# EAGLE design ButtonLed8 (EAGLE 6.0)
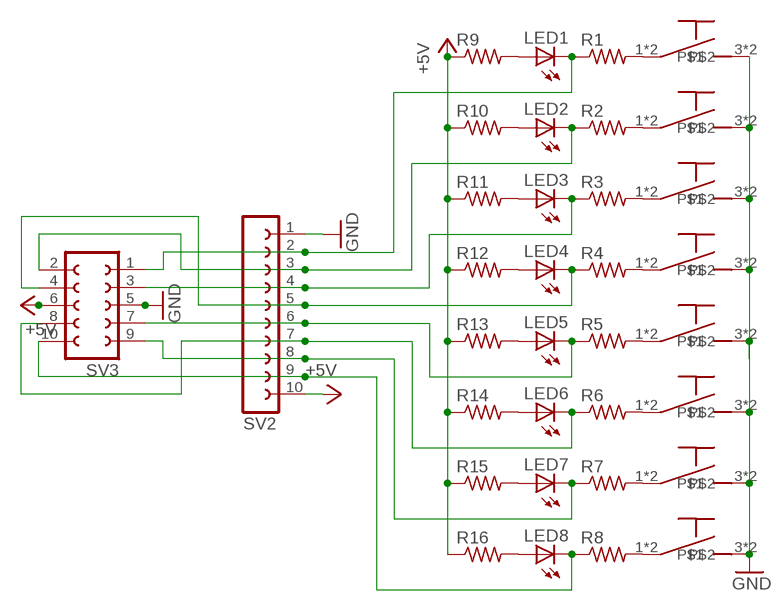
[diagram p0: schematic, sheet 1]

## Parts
LED1  LED3MM  [LED3MM]
LED2  LED3MM  [LED3MM]
LED3  LED3MM  [LED3MM]
LED4  LED3MM  [LED3MM]
LED5  LED3MM  [LED3MM]
LED6  LED3MM  [LED3MM]
LED7  LED3MM  [LED3MM]
LED8  LED3MM  [LED3MM]
R1  R-US_0204/7  [0204/7]
R2  R-US_0204/7  [0204/7]
R3  R-US_0204/7  [0204/7]
R4  R-US_0204/7  [0204/7]
R5  R-US_0204/7  [0204/7]
R6  R-US_0204/7  [0204/7]
R7  R-US_0204/7  [0204/7]
R8  R-US_0204/7  [0204/7]
R9  R-US_0204/7  [0204/7]
R10  R-US_0204/7  [0204/7]
R11  R-US_0204/7  [0204/7]
R12  R-US_0204/7  [0204/7]
R13  R-US_0204/7  [0204/7]
R14  R-US_0204/7  [0204/7]
R15  R-US_0204/7  [0204/7]
R16  R-US_0204/7  [0204/7]
SV2  FE10-1  [FE10]
SV3  FE05-2  [FE05-2]
U$1  BUTTON  [SPARKFUN_TACTILE-PTH]
U$2  BUTTON  [SPARKFUN_TACTILE-PTH]
U$3  BUTTON  [SPARKFUN_TACTILE-PTH]
U$4  BUTTON  [SPARKFUN_TACTILE-PTH]
U$5  BUTTON  [SPARKFUN_TACTILE-PTH]
U$6  BUTTON  [SPARKFUN_TACTILE-PTH]
U$7  BUTTON  [SPARKFUN_TACTILE-PTH]
U$8  BUTTON  [SPARKFUN_TACTILE-PTH]

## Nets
+5V: R9.1 R10.1 R11.1 R12.1 R13.1 R14.1 R15.1 R16.1 SV2.10 SV3.6
GND: SV2.1 SV3.5 U$1.3 U$1.4 U$2.3 U$2.4 U$3.3 U$3.4 U$4.3 U$4.4 U$5.3 U$5.4 U$6.3 U$6.4 U$7.3 U$7.4 U$8.3 U$8.4
N$1: R1.2 U$1.1 U$1.2
N$2: R2.2 U$2.1 U$2.2
N$3: R4.2 U$4.1 U$4.2
N$4: R5.2 U$5.1 U$5.2
N$5: R6.2 U$6.1 U$6.2
N$6: R7.2 U$7.1 U$7.2
N$7: R8.2 U$8.1 U$8.2
N$8: LED1.K(C) R1.1 SV2.2 SV3.1
N$10: LED3.K(C) R3.1 SV2.4 SV3.3
N$11: LED4.K(C) R4.1 SV2.5 SV3.4
N$12: LED5.K(C) R5.1 SV2.6 SV3.7
N$13: LED6.K(C) R6.1 SV2.7 SV3.8
N$14: LED7.K(C) R7.1 SV2.8 SV3.9
N$15: LED8.K(C) R8.1 SV2.9 SV3.10
N$16: R3.2 U$3.1 U$3.2
N$17: LED1.A R9.2
N$18: LED2.A R10.2
N$19: LED3.A R11.2
N$20: LED4.A R12.2
N$21: LED5.A R13.2
N$22: LED6.A R14.2
N$23: LED7.A R15.2
N$24: LED8.A R16.2
N$25: LED2.K(C) R2.1 SV2.3 SV3.2

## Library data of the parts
LED1-LED8 = led:LED: LED
R1-R16 = resistor:R-US_: RESISTOR, American symbol
SV2 = con-lsta:FE10-1: FEMALE HEADER; OC_FARNELL: unknown; OC_NEWARK: unknown
SV3 = con-lsta:FE05-2: FEMALE HEADER; OC_FARNELL: unknown; OC_NEWARK: unknown
U$1-U$8 = Iodph:BUTTON

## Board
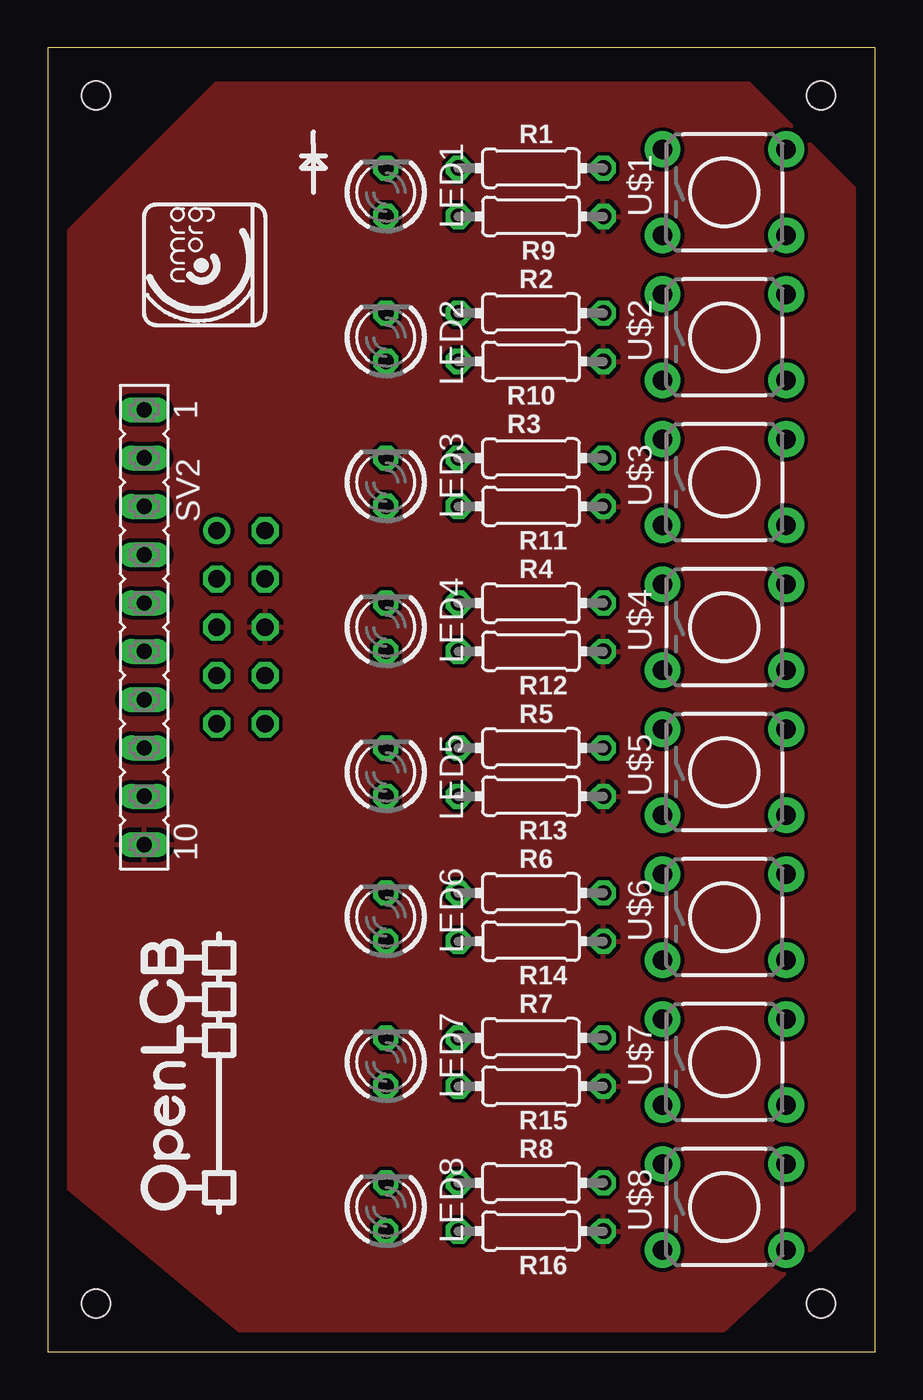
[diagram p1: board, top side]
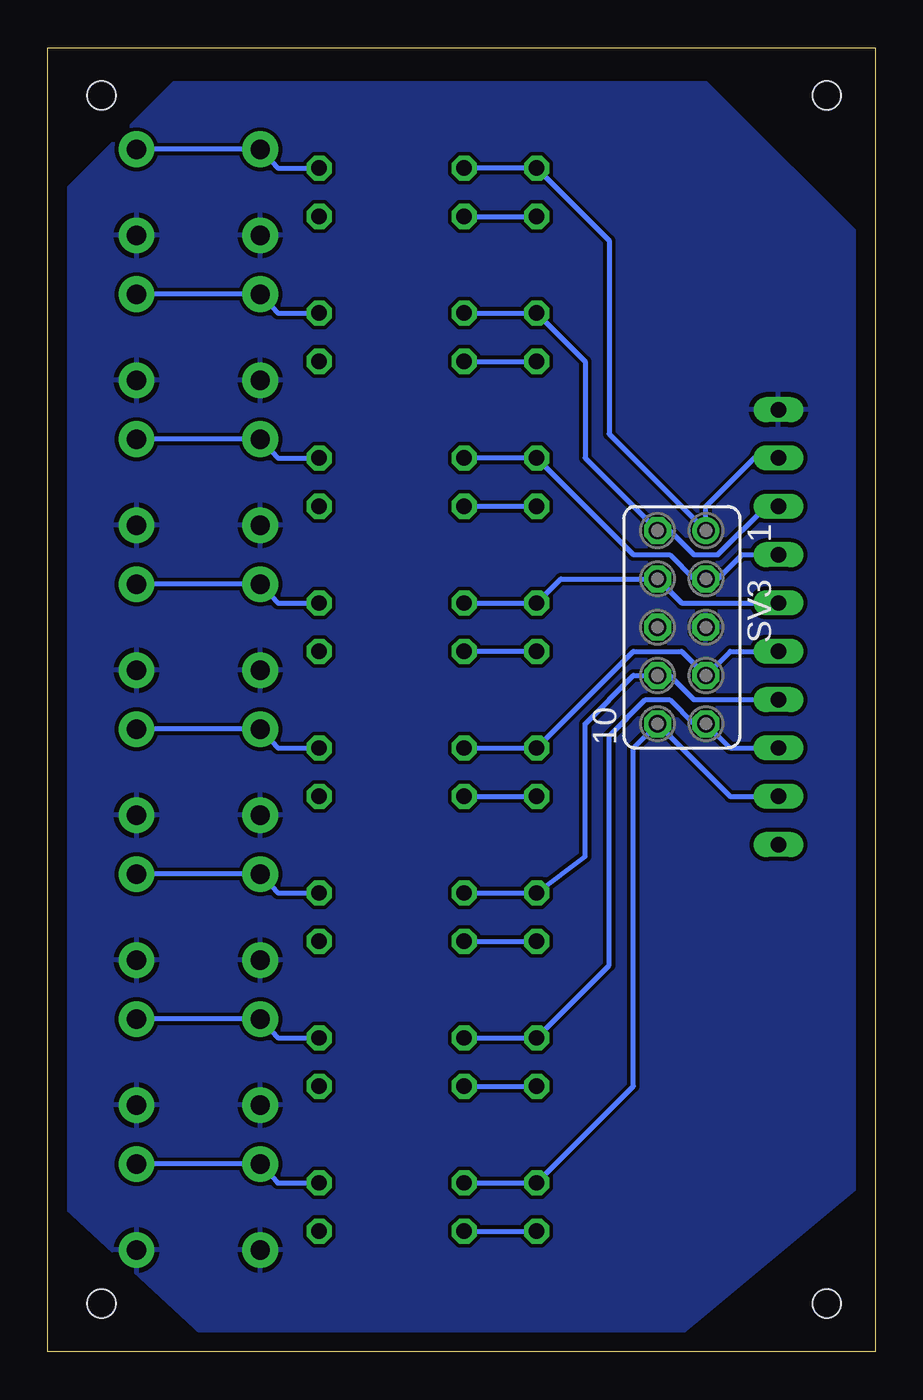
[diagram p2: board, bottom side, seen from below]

Size 43.48 x 68.57 mm. Coordinates in mm from the lower left corner, seen from the top.
Outline: 0,0 43.48,0 43.48,68.57 0,68.57 0,0
Copper layers (1*16): Top 0.035mm / dielectric 1.5mm / Bottom 0.035mm
Design rules: minimum track width 10mil, minimum drill 24mil, track to track 8mil, track to pad 8mil, pad to pad 8mil, via to via 8mil, smd to smd 8mil, copper to edge 40mil, drill to drill 8mil, minimum pad ring 10mil, minimum via ring 8mil, stop-mask expansion 4mil, vias tented up to drill 0mil, thermal gap 10mil
Holes 1.5 mm at 40.64,66.04 2.54,66.04 2.54,2.54 40.64,2.54

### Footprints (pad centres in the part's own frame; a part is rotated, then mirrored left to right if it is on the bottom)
LED3MM = drill 0.813 octagon: A -1.27,0; K 1.27,0
0204/7 = drill 0.813 octagon: 1 -3.81,0; 2 3.81,0
FE10 = drill 0.813 long: 1 -11.43,0; 2 -8.89,0; 3 -6.35,0; 4 -3.81,0; 5 -1.27,0; 6 1.27,0; 7 3.81,0; 8 6.35,0; 9 8.89,0; 10 11.43,0
FE05-2 = drill 0.914: 1 -5.08,1.27 | drill 0.914 octagon: 2 -5.08,-1.27; 3 -2.54,1.27; 4 -2.54,-1.27; 5 0,1.27; 6 0,-1.27; 7 2.54,1.27; 8 2.54,-1.27; 9 5.08,1.27; 10 5.08,-1.27
SPARKFUN_TACTILE-PTH = drill 1.016 pad 1.88: 1 -3.251,2.261; 2 3.251,2.261; 3 -3.251,-2.261; 4 3.251,-2.261

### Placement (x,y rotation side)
LED1  17.78,60.96 90 top
LED2  17.78,53.34 90 top
LED3  17.78,45.72 90 top
LED4  17.78,38.1 90 top
LED5  17.78,30.48 90 top
LED6  17.78,22.86 90 top
LED7  17.78,15.24 90 top
LED8  17.78,7.62 90 top
R1  25.4,62.23 0 top
R2  25.4,54.61 0 top
R3  25.4,46.99 0 top
R4  25.4,39.37 0 top
R5  25.4,31.75 0 top
R6  25.4,24.13 0 top
R7  25.4,16.51 0 top
R8  25.4,8.89 0 top
R9  25.4,59.69 180 top
R10  25.4,52.07 180 top
R11  25.4,44.45 180 top
R12  25.4,36.83 180 top
R13  25.4,29.21 180 top
R14  25.4,21.59 180 top
R15  25.4,13.97 180 top
R16  25.4,6.35 180 top
SV2  5.08,38.1 270 top
SV3  10.16,38.1 270 bottom
U$1  35.56,60.96 0 top
U$2  35.56,53.34 0 top
U$3  35.56,45.72 0 top
U$4  35.56,38.1 0 top
U$5  35.56,30.48 0 top
U$6  35.56,22.86 0 top
U$7  35.56,15.24 0 top
U$8  35.56,7.62 0 top
U$9  [OPENLCB_LOGOV]  10.16,6.99 90 top
U$10  [NMRA_ORG_SMALL]  11.43,53.98 90 top

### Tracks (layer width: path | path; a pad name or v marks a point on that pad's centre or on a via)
+5V
  pour Top: 8.89,66.67 36.83,66.67 43.18,60.33 43.18,8.26 34.29,0 11.43,0 0,9.53 0,57.78
GND
  pour Bottom: 8.89,66.67 36.83,66.67 43.18,60.33 43.18,8.26 34.29,0 11.43,0 0,9.53 0,57.78
N$1
  Bottom 0.254: R1.2 31.39,62.23 U$1.1 U$1.2
N$2
  Bottom 0.254: R2.2 31.39,54.61 U$2.1 U$2.2
N$3
  Bottom 0.254: R4.2 31.39,39.37 U$4.1 U$4.2
N$4
  Bottom 0.254: R5.2 31.39,31.75 U$5.1 U$5.2
N$5
  Bottom 0.254: R6.2 31.39,24.13 U$6.1 U$6.2
N$6
  Bottom 0.254: R7.2 31.39,16.51 U$7.1 U$7.2
N$7
  Bottom 0.254: R8.2 31.39,8.89 U$8.1 U$8.2
N$8
  Bottom 0.254: R1.1 LED1.K 13.97,58.42 13.97,48.26 SV3.1 8.89,44.45 6.35,46.99 SV2.2
N$10
  Bottom 0.254: R3.1 LED3.K 12.7,41.91 10.79,41.91 9.53,40.64 SV3.3 8.26,40.64 6.99,41.91 SV2.4
N$11
  Bottom 0.254: R4.1 LED4.K 16.51,40.64 SV3.4 10.16,39.37 SV2.5
N$12
  Bottom 0.254: R5.1 LED5.K 12.7,36.83 10.16,36.83 SV3.7 7.62,36.83 SV2.6
N$13
  Bottom 0.254: R6.1 LED6.K 15.24,26.04 15.24,33.02 12.7,35.56 SV3.8 10.79,35.56 9.53,34.29 SV2.7
N$14
  Bottom 0.254: R7.1 LED7.K 13.97,20.32 13.97,32.38 12.06,34.29 10.79,34.29 9.53,33.02 SV3.9 7.62,31.75 SV2.8
N$15
  Bottom 0.254: R8.1 LED8.K 12.7,13.97 12.7,31.75 SV3.10 7.62,29.21 SV2.9
N$16
  Bottom 0.254: R3.2 31.39,46.99 U$3.1 U$3.2
N$17
  Bottom 0.254: R9.2 LED1.A
N$18
  Bottom 0.254: R10.2 LED2.A
N$19
  Bottom 0.254: LED3.A R11.2
N$20
  Bottom 0.254: LED4.A R12.2
N$21
  Bottom 0.254: R13.2 LED5.A
N$22
  Bottom 0.254: R14.2 LED6.A
N$23
  Bottom 0.254: R15.2 LED7.A
N$24
  Bottom 0.254: R16.2 LED8.A
N$25
  Bottom 0.254: R2.1 LED2.K 15.24,52.07 15.24,46.99 SV3.2 10.79,43.18 9.53,41.91 8.26,41.91 5.71,44.45 SV2.3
